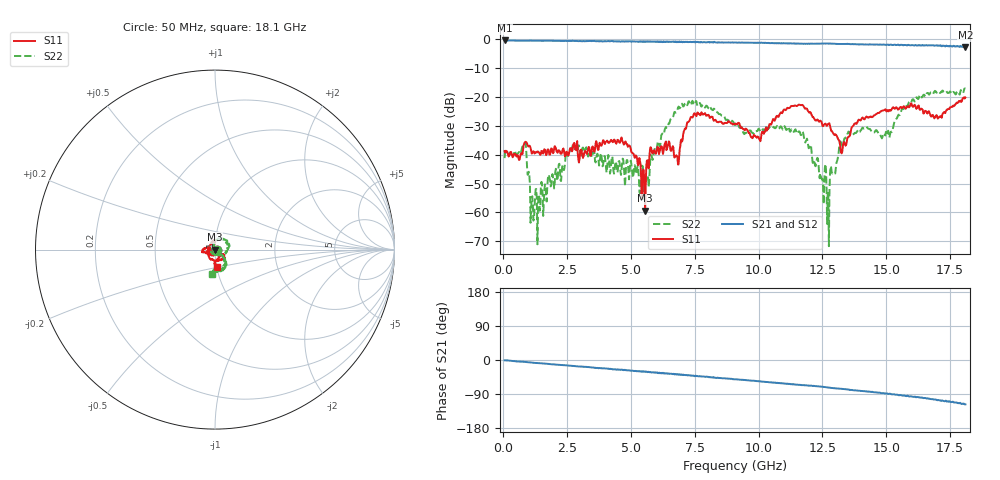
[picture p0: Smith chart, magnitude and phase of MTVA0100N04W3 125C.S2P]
! Network Analyzer HP8720D.06.14 Serial No. US36140669
! 17 Jan 2005  10:55:03
! Frequency  S11  S21  S12  S22
# HZ  S  DB R 50
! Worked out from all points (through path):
!   801 points, 50 MHz to 18.1 GHz, reference 50 ohm
!   highest |S21| = -0.52 dB at 50 MHz (marker M1); lowest = -2.9 dB at 18.1 GHz (marker M2)
!   group delay of S21, straight-line fit = 16.9 ps
!   lowest |S11| = -59.4 dB at 5.555 GHz (marker M3), VSWR 1.00, Z = 49.9 + j0.0275 ohm
!   |S11| at or under -10 dB: start of sweep to end of sweep
!   |S22| runs from -71.6 to -17.1 dB; largest |S21 - S12| = 0.027
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5e7  -38.78 -16.3  -0.52 -0.8  -0.56 -1.1  -41.19 -14.9
8.17125e8  -36.11 14.2  -0.61 -4.9  -0.59 -5.3  -36.98 -38.6
1.155562e9  -38.96 -6.1  -0.58 -7.0  -0.59 -7.4  -57.02 -47.0
2.66725e9  -38.31 13.8  -0.67 -15.3  -0.66 -15.6  -38.59 117.7
3.073375e9  -39.08 45.4  -0.74 -17.6  -0.70 -17.9  -38.70 -82.0
4.697875e9  -35.88 35.4  -0.77 -26.2  -0.81 -26.3  -41.85 76.1
5.2845e9  -43.63 95.3  -0.93 -30.0  -0.89 -30.1  -45.18 0.0
5.487562e9  -45.18 136.8  -0.78 -30.3  -0.80 -30.8  -49.06 -88.3
5.55525e9  -59.41 165.1  -0.83 -30.4  -0.81 -30.9  -50.46 -14.1
6.074188e9  -37.78 -129.1  -0.99 -34.7  -0.99 -34.6  -35.57 122.4
6.796188e9  -40.40 -154.6  -1.12 -38.3  -1.06 -38.2  -25.26 75.9
7.202312e9  -28.83 97.8  -0.96 -40.2  -1.02 -40.6  -22.91 42.1
9.075e9  -29.35 -166.8  -1.26 -50.7  -1.24 -51.0  -29.77 -64.4
1.000006e10  -33.98 -163.8  -1.33 -56.2  -1.32 -56.3  -31.02 -65.3
1.164712e10  -22.89 -169.7  -1.62 -65.7  -1.60 -66.0  -33.19 -155.0
1.209838e10  -26.70 -151.4  -1.60 -68.4  -1.63 -68.5  -41.30 152.2
1.273012e10  -29.46 -104.3  -1.62 -72.7  -1.60 -73.3  -53.11 -136.3
1.345212e10  -35.48 -110.5  -1.73 -77.2  -1.73 -77.6  -33.71 -48.4
1.509919e10  -24.98 -103.3  -2.09 -89.5  -1.98 -89.8  -33.55 -64.5
1.597912e10  -22.27 -48.4  -2.15 -96.0  -2.19 -97.2  -22.01 -45.9
1.708469e10  -26.91 -52.4  -2.32 -106.6  -2.19 -107.2  -18.45 -78.2
1.81e10  -20.27 -82.6  -2.88 -117.0  -2.77 -117.6  -17.18 -96.1
